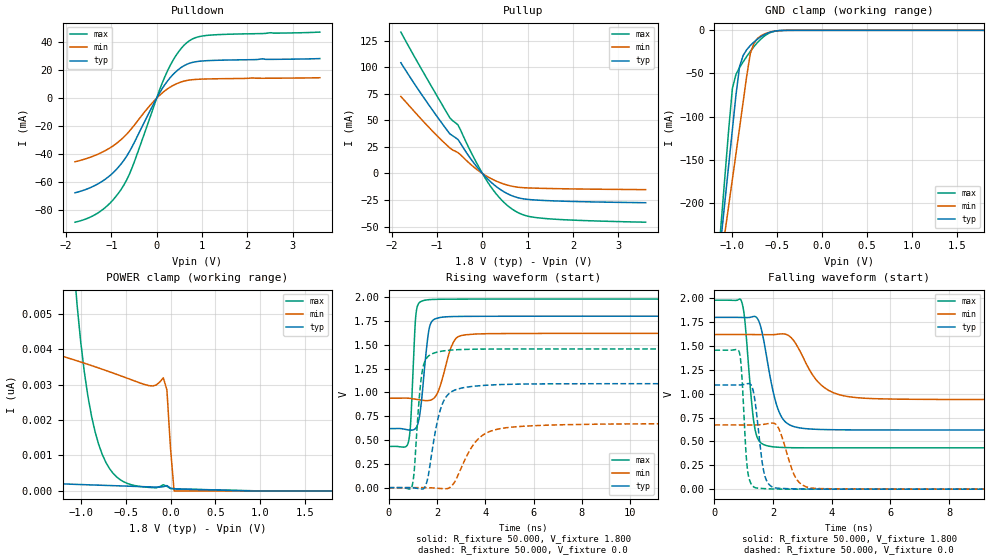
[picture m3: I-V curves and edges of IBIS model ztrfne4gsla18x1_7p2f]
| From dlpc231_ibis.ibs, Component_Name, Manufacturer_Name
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| Model ztrfne4gsla18x1_7p2f
[Model] ztrfne4gsla18x1_7p2f
Model_type I/O
Polarity   Non-Inverting
Enable   Active-High
Vinl =  0.540V
Vinh =  1.260V
Vref = 0.000V
Rref = 0.50k
Cref = 50.00pF
Vmeas = 0.90V
C_comp   2.433pF   2.338pF   2.581pF
C_comp_pullup   0.677pF   0.575pF   0.876pF
C_comp_pulldown   0.677pF   0.575pF   0.876pF
[Temperature Range]   25.000   0.125k   -40.000
[Voltage Range]   1.800V   1.620V   1.980V
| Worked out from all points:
|   slope of the pulldown table from 0 to 0.27 V, typ, clamps not added: 19.9 ohm
|   slope of the pullup table from 0 to 0.27 V, typ, clamps not added: 24.3 ohm
|   GND clamp passes 1 mA (typ) near -0.53 V on its own axis
|   rising waveform, R_fixture 50.000, V_fixture 1.800: 20-80 % time 279ps typ, 461ps min, 163ps max; typ from 0.62 V to 1.8 V
|   rising waveform, R_fixture 50.000, V_fixture 0.0: 20-80 % time 516ps typ, 949ps min, 266ps max; typ from 0 V to 1.09 V
|   falling waveform, R_fixture 50.000, V_fixture 1.800: 20-80 % time 470ps typ, 851ps min, 260ps max; typ from 1.8 V to 0.62 V
|   falling waveform, R_fixture 50.000, V_fixture 0.0: 20-80 % time 257ps typ, 432ps min, 158ps max; typ from 1.09 V to 0 V
[Pulldown]
-1.8V     -67.78mA   -45.55mA   -88.87mA
-1.2V     -59.54mA   -38.67mA   -80.11mA
-960mV    -53.44mA   -34.19mA   -72.85mA
-720mV    -44.39mA   -27.75mA   -62.11mA
-540mV    -34.73mA   -21.28mA   -49.74mA
-120mV    -7.451mA   -4.22mA    -11.37mA
180mV     9.688mA    5.261mA    15.31mA
420mV     18.87mA    10.09mA    30.28mA
660mV     24.23mA    12.68mA    39.65mA
900mV     26.34mA    13.56mA    43.85mA
1.2V      27.05mA    13.87mA    45.28mA
3.6V      28.41mA    14.68mA    47.41mA
[Pullup]
-1.8V     104.2mA    72.43mA    133mA
-1.26V    69.23mA    46.97mA    91.9mA
-720mV    37.3mA     24.04mA    52.35mA
-540mV    31.98mA    19.65mA    45.69mA
-300mV    16.31mA    10.05mA    24.1mA
-60mV     2.962mA    1.758mA    4.549mA
240mV     -10.09mA   -5.893mA   -15.76mA
420mV     -15.8mA    -9.168mA   -24.87mA
600mV     -20mA      -11.49mA   -31.8mA
900mV     -23.85mA   -13.35mA   -38.91mA
1.26V     -25.17mA   -13.9mA    -41.85mA
3.6V      -27.51mA   -15.2mA    -45.81mA
[GND_clamp]
-1.8V     -927mA     -775.7mA   -1.101A
-1.16V    -275.3mA   -291.3mA   -268.1mA
-1.12V    -235.1mA   -261.5mA   -216.5mA
-1.08V    -194.9mA   -231.7mA   -164.9mA
-1V       -114.9mA   -172.5mA   -67.23mA
-920mV    -41.99mA   -112.9mA   -43.08mA
-880mV    -29.06mA   -82.77mA   -36.47mA
-800mV    -17.56mA   -26.87mA   -24.31mA
-760mV    -13.55mA   -15.08mA   -18.89mA
-680mV    -7.158mA   -6.178mA   -9.822mA
-440mV    -133.7uA   -176.5uA   -112.6uA
1.8V      0A         0A         0A
[POWER_clamp]
-1.8V     288.6pA    4.231nA    140.6nA
-1.08V    187.2pA    3.703nA    6.484nA
-1.04V    183.6pA    3.671nA    5.234nA
-960mV    176.5pA    3.605nA    3.359nA
-840mV    166pA      3.504nA    1.668nA
-720mV    155.7pA    3.399nA    806.1pA
-560mV    142pA      3.253nA    315.8pA
-200mV    111.6pA    2.962nA    92.54pA
-80mV     117.3pA    3.191nA    175.1pA
-40mV     151.6pA    2.851nA    129.2pA
40mV      60.08pA    0A         58.67pA
1.8V      0A         0A         0A
[Ramp]
dV/dt_r   0.655/0.518n   0.404/0.945n   0.874/0.270n
dV/dt_f   0.708/0.474n   0.409/0.857n   0.928/0.264n
R_load = 50.000
[Rising Waveform]
R_fixture= 50.000
V_fixture= 1.800
V_fixture_min= 1.620
V_fixture_max= 1.980
0s        620.3mV    939mV      433.1mV
829ps     606.4mV    939.1mV    489.1mV
919ps     604.2mV    936.5mV    711mV
1.12ns    623.1mV    928.4mV    1.788V
1.372ns   937.7mV    918.5mV    1.958V
1.674ns   1.664V     915.4mV    1.974V
2.064ns   1.783V     1.019V     1.978V
2.604ns   1.796V     1.484V     1.979V
3.055ns   1.798V     1.6V       1.98V
15ns      1.8V       1.62V      1.98V
[Rising Waveform]
R_fixture= 50.000
V_fixture= 0.0
V_fixture_min= 0.0
V_fixture_max= 0.0
0s        0V         0V         0V
969ps     -610.5uV   576.2uV    12.64mV
1.379ns   -14.01mV   449.6uV    1.202V
1.602ns   79.4mV     -159.1uV   1.369V
1.832ns   437.5mV    -2.406mV   1.409V
2.33ns    934.2mV    -10.91mV   1.438V
3.13ns    1.051V     278.3mV    1.451V
3.85ns    1.072V     543.2mV    1.455V
4.86ns    1.084V     629.2mV    1.456V
15ns      1.092V     672.6mV    1.456V
[Falling Waveform]
R_fixture= 50.000
V_fixture= 1.800
V_fixture_min= 1.620
V_fixture_max= 1.980
0s        1.8V       1.62V      1.98V
931ps     1.799V     1.62V      1.962V
1.041ns   1.798V     1.62V      1.751V
1.351ns   1.81V      1.62V      684.5mV
1.725ns   1.482V     1.619V     461.3mV
2.205ns   807.7mV    1.625V     438.7mV
2.848ns   645.3mV    1.485V     433.8mV
3.638ns   625.3mV    1.091V     433.2mV
4.589ns   621.3mV    968.3mV    433.2mV
15ns      620.3mV    939mV      433.1mV
[Falling Waveform]
R_fixture= 50.000
V_fixture= 0.0
V_fixture_min= 0.0
V_fixture_max= 0.0
0s        1.092V     672.9mV    1.456V
851ps     1.092V     672.7mV    1.431V
921ps     1.093V     672.7mV    1.249V
1.121ns   1.105V     672.6mV    217.7mV
1.396ns   892.1mV    673mV      15.1mV
1.686ns   178.5mV    679.4mV    5.95mV
2.058ns   14.05mV    686.9mV    1.776mV
2.779ns   3.042mV    114.5mV    180.6uV
3.308ns   1.176mV    11.32mV    35.67uV
15ns      0V         0V         0V
